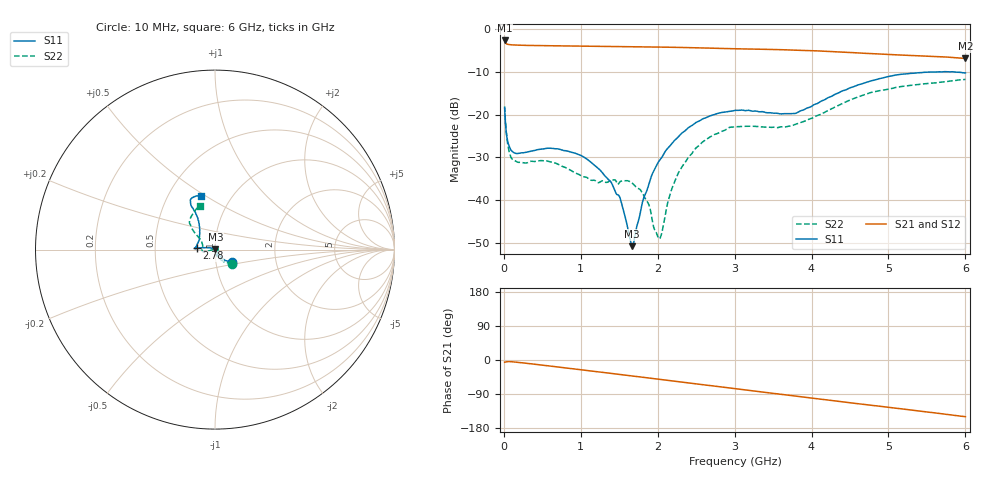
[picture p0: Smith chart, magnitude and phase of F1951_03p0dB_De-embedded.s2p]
! Integrated Device Technology
! Corporate Headquarters
! 6024 Silver Creek Valley Road
! San Jose, CA 95138  USA
! Phone:  1-408-284-8200
! Toll Free:  1-800-223-1366
! Webpage:  http://www.idt.com/
! Timing and RF Division
! 515 Groton Road, Suite 102
! Westford, MA 01886-6024
! Device:  F1951
! Description: 6-bit 0.5 dB Digital Step Attenuator
! Frequency:  100.0 -  4000.00 MHz
! Package:  4x4 mm Thin QFN Plastic Package: 24 pin
! Ports:  2 RF, 6 DC
!  Pin  1  = NC
!  Pin  2  = RF1  =  Port 1
!  Pin  3  = GND
!  Pin  4  = NC
!  Pin  5  = Serial Data Out (SDO)
!  Pin  6  = NC
!  Pin  7  = Reset Bar ( RSTb)
!  Pin  8  = Clock (CLK)
!  Pin  9  = Chip Select Bar (CSb)
!  Pin 10  = NC
!  Pin 11  = Serial Data In (SDI)
!  Pin 12  = NC
!  Pin 13  = NC
!  Pin 14  = VDD
!  Pin 15  = NC
!  Pin 16  = GND
!  Pin 17  = RF2  =  Port 2
!  Pin 18  = NC
!  Pin 19  = GND
!  Pin 20  = GND
!  Pin 21  = GND
!  Pin 22  = GND
!  Pin 23  = GND
!  Pin 24  = GND
! State:  6
! Atten State:  3.0 dB
! Voltage:  +3.30 Volts
! Current:  0.475 mA
! Data:  The device was measured on a F195X evaluation board which has
!  individual transmission lines to the RF pins.  Data was collected
!  de-embedded using a Automatic Fixture Removal [AFR] (Keysight Technologies).
!  The reference plane is the edge of the package pin.
! Misc:  Lot Code  1225BCA
!  Action Tracker AT0399
! Date Measured:  2018-09-13
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# GHz S dB R 50
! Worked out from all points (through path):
!   600 points, 10 MHz to 6 GHz, reference 50 ohm
!   highest |S21| = -2.64 dB at 10 MHz (marker M1); lowest = -6.8 dB at 6 GHz (marker M2)
!   group delay of S21, straight-line fit = 68.7 ps
!   lowest |S11| = -50.8 dB at 1.67 GHz (marker M3), VSWR 1.01, Z = 50.2 + j0.202 ohm
!   |S11| at or under -10 dB: start of sweep to 5.631 GHz; 5.668 GHz to 5.705 GHz (36.51 MHz wide, 0.642 % of centre); 5.847 GHz to end of sweep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
!   |S22| runs from -49.1 to -11.8 dB; largest |S21 - S12| = 0.00078
!   S11 on the Smith chart (normalised r, x): 10 MHz: 1.20, -0.17; 2.78 GHz: 0.81, +0.01; 6 GHz: 0.73, +0.48
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0.01  -18.52 -36.8  -2.64 -5.9  -2.64 -5.9  -18.08 -39.0
0.07  -27.37 -52.2  -3.61 -4.2  -3.62 -4.2  -28.83 -66.7
0.13  -28.92 -57.4  -3.70 -5.1  -3.70 -5.1  -30.67 -71.7
0.63  -27.93 -73.4  -3.89 -16.7  -3.89 -16.7  -31.16 -79.0
1.01  -29.64 -60.0  -3.97 -26.0  -3.97 -26.0  -34.38 -48.7
1.4  -36.02 -33.9  -4.04 -35.5  -4.04 -35.5  -35.29 5.6
1.52  -40.11 -18.9  -4.06 -38.4  -4.07 -38.4  -35.62 20.4
1.67  -50.83 44.4  -4.09 -42.2  -4.09 -42.2  -36.08 28.4
1.87  -37.21 150.2  -4.14 -47.3  -4.15 -47.2  -40.54 40.3
1.96  -32.83 156.4  -4.17 -49.5  -4.17 -49.5  -46.95 59.6
2.01  -31.08 160.2  -4.18 -50.8  -4.19 -50.8  -48.79 110.0
2.05  -30.13 161.6  -4.20 -51.8  -4.20 -51.8  -47.93 151.1
2.17  -27.11 165.6  -4.24 -54.8  -4.24 -54.8  -38.12 -176.9
2.29  -24.79 168.8  -4.28 -57.9  -4.28 -57.9  -32.98 -170.3
2.51  -21.75 173.4  -4.36 -63.4  -4.37 -63.4  -27.64 -167.2
2.78  -19.72 176.1  -4.49 -70.2  -4.50 -70.2  -24.42 -169.3
3.01  -19.01 177.3  -4.58 -75.8  -4.59 -75.8  -22.85 -174.4
3.76  -19.77 147.9  -4.90 -94.5  -4.90 -94.5  -22.49 157.7
4.01  -17.94 131.9  -5.04 -100.8  -5.04 -100.8  -20.86 147.9
4.56  -13.37 118.1  -5.52 -114.3  -5.52 -114.3  -16.17 139.4
5.01  -11.06 118.5  -5.94 -125.0  -5.95 -125.0  -14.05 134.6
6  -10.24 104.3  -6.84 -149.5  -6.85 -149.6  -11.76 109.4
